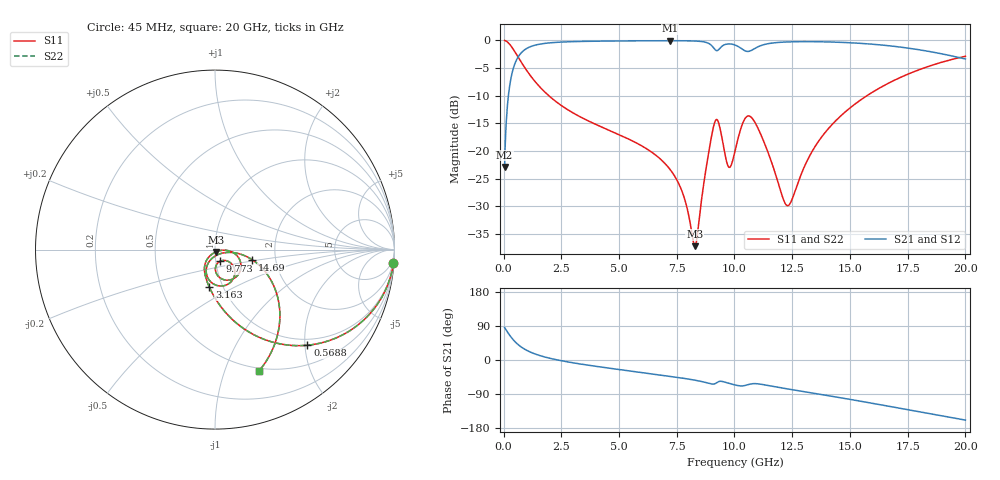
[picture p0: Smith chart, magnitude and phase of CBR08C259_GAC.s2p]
! S-parameter model data by Modelithics Inc.  support@modelithics.com 813-866-6335  Tampa FL USA
! S-Parameter data specifications:
! Substrate: 20-mil Rogers 4350B, substrate thickness, H=0.508mm, Dielectric constant, Er=3.75
! PCB Mounting Pad Footprint: Pad width, PadW=1.45mm , Pad length, PadL=1mm , Pad gap, PadG (edge-to-edge)=0.6mm , Reference planes=2.6mm apart
#  GHz  S  MA  R 50
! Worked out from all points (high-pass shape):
!   801 points, 45 MHz to 20 GHz, reference 50 ohm
!   highest |S21| = -0.07 dB at 7.204 GHz (marker M1); lowest = -22.9 dB at 45 MHz (marker M2)
!   |S21| within 3 dB of the highest: 621.4 MHz to 19.68 GHz (19.06 GHz wide, 188 % of centre)
!   lowest |S11| = -37.2 dB at 8.276 GHz (marker M3), VSWR 1.03, Z = 50.4 - j1.31 ohm
!   |S11| at or under -10 dB: 1.957 GHz to 15.74 GHz (13.78 GHz wide, 156 % of centre)
!   |S22| runs from -37.2 to 0.0 dB; largest |S21 - S12| = 0
!   S11 on the Smith chart (normalised r, x): 45 MHz: 1, -26; 568.8 MHz: 0.87, -2.05; 3.163 GHz: 0.86, -0.38; 9.773 GHz: 1.05, -0.14; 14.69 GHz: 1.51, -0.18; 20 GHz: 0.47, -1.32
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0.045  0.9974 -4.4  0.07171 85.6  0.07171 85.6  0.9974 -4.4
0.269494  0.9184 -25.1  0.3951 64.9  0.3951 64.9  0.9184 -25.1
0.568819  0.741 -46.0  0.6708 44.0  0.6708 44.0  0.741 -46.0
0.942975  0.5567 -62.4  0.8297 27.5  0.8297 27.5  0.5567 -62.4
1.416906  0.4117 -75.1  0.91 14.8  0.91 14.8  0.4117 -75.1
3.162969  0.2119 -98.5  0.9752 -9.0  0.9752 -9.0  0.2119 -98.5
3.387462  0.2001 -100.6  0.9776 -11.1  0.9776 -11.1  0.2001 -100.6
6.704981  0.08767 -126.5  0.9918 -38.9  0.9918 -38.9  0.08767 -126.5
7.203856  0.06837 -129.1  0.9922 -43.0  0.9922 -43.0  0.06837 -129.1
7.777563  0.04045 -127.9  0.9912 -48.1  0.9912 -48.1  0.04045 -127.9
8.276438  0.01379 -70.5  0.9859 -53.2  0.9859 -53.2  0.01379 -70.5
9.149469  0.1828 -39.2  0.8288 -62.7  0.8288 -62.7  0.1828 -39.2
9.324075  0.177 -72.6  0.8276 -56.8  0.8276 -56.8  0.177 -72.6
9.773062  0.07102 -66.3  0.9282 -61.8  0.9282 -61.8  0.07102 -66.3
10.0225  0.09976 -41.4  0.9073 -65.9  0.9073 -65.9  0.09976 -41.4
10.39666  0.1863 -55.3  0.8163 -68.0  0.8163 -68.0  0.1863 -55.3
10.74587  0.1997 -87.3  0.8138 -62.8  0.8138 -62.8  0.1997 -87.3
12.29238  0.03203 -66.6  0.9672 -76.3  0.9672 -76.3  0.03203 -66.6
13.36496  0.09933 -9.5  0.9727 -87.1  0.9727 -87.1  0.09933 -9.5
14.68698  0.2153 -15.3  0.9577 -100.6  0.9577 -100.6  0.2153 -15.3
16.68248  0.4111 -34.4  0.8936 -122.1  0.8936 -122.1  0.4111 -34.4
20  0.7178 -69.9  0.6776 -158.6  0.6776 -158.6  0.7178 -69.9
